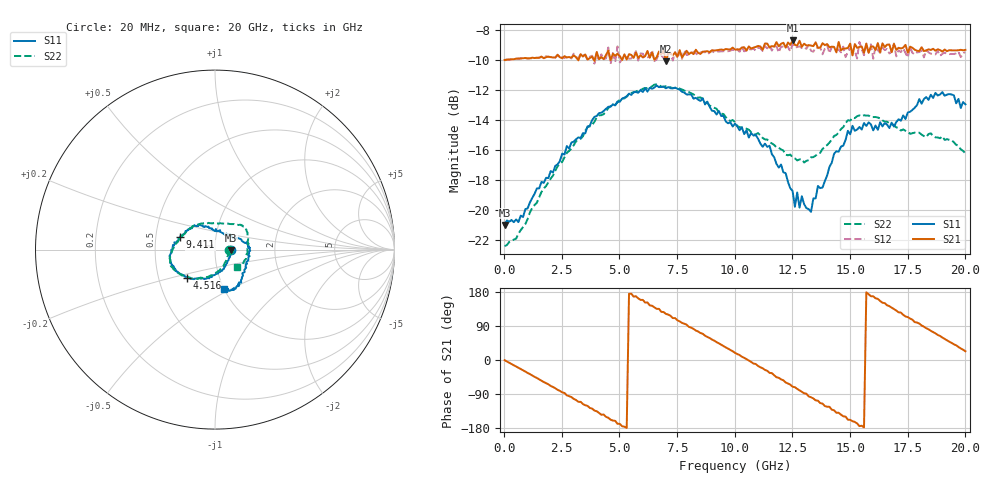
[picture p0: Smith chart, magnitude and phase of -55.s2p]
!Agilent Technologies,N5230A,US43500223,A.07.50.48
!Agilent N5230A: A.07.50.48
!Date: Saturday, October 10, 2015 17:03:50
!Correction: S11(Full 2 Port(1,2))
!S21(Full 2 Port(1,2))
!S12(Full 2 Port(1,2))
!S22(Full 2 Port(1,2))
!S2P File: Measurements: S11, S21, S12, S22:
# Hz S  RI  R 50
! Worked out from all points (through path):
!   201 points, 20 MHz to 20 GHz, reference 50 ohm
!   highest |S21| = -8.68 dB at 12.51 GHz (marker M1); lowest = -10.1 dB at 7.013 GHz (marker M2)
!   group delay of S21, straight-line fit = 96.8 ps
!   lowest |S11| = -21.0 dB at 20 MHz (marker M3), VSWR 1.20, Z = 59.8 - j0.339 ohm
!   |S11| at or under -10 dB: start of sweep to end of sweep
!   |S22| runs from -22.4 to -11.6 dB; largest |S21 - S12| = 0.034
!   S11 on the Smith chart (normalised r, x): 20 MHz: 1.20, -0.01; 4.516 GHz: 0.70, -0.23; 9.411 GHz: 0.67, +0.10; 20 GHz: 1.00, -0.46
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2e7  0.0892 -0.00281  0.3171 -0.00319  0.316 -0.00303  0.0758 -0.00311
1.8182e9  0.0285 -0.1251  0.1564 -0.2835  0.1554 -0.2872  0.0192 -0.1189
3.4166e9  -0.0786 -0.1627  -0.1436 -0.2921  -0.155 -0.2898  -0.0822 -0.1563
4.5155e9  -0.1551 -0.1579  -0.302 -0.1575  -0.3102 -0.1603  -0.1563 -0.1535
4.6154e9  -0.1619 -0.1509  -0.2926 -0.1219  -0.2871 -0.109  -0.1603 -0.1543
5.7143e9  -0.2166 -0.1205  -0.3285 0.0687  -0.3322 0.0691  -0.216 -0.1235
6.7133e9  -0.2477 -0.0698  -0.2394 0.2389  -0.2319 0.2411  -0.2459 -0.0903
7.013e9  -0.2485 -0.0579  -0.1649 0.2674  -0.1692 0.2797  -0.249 -0.0722
8.3117e9  -0.2365 0.0153  0.0729 0.3351  0.0835 0.3234  -0.2406 -0.011
9.4106e9  -0.1947 0.068  0.2621 0.2221  0.2635 0.2131  -0.2038 0.0506
1.001e10  -0.1641 0.1041  0.3249 0.111  0.3233 0.1025  -0.1787 0.0816
1.14086e10  -0.0912 0.1348  0.3157 -0.1717  0.2967 -0.1791  -0.1009 0.1393
1.25075e10  -0.0186 0.1145  0.1229 -0.3472  0.1184 -0.3383  -0.0297 0.1471
1.26074e10  0.00134 0.1026  0.1113 -0.3382  0.089 -0.3373  -0.0252 0.1468
1.34066e10  0.0636 0.0891  -0.0702 -0.3456  -0.0718 -0.33  0.0369 0.1457
1.45055e10  0.1486 0.0496  -0.2758 -0.2376  -0.2603 -0.2242  0.118 0.1382
1.53047e10  0.185 0.0164  -0.3397 -0.0759  -0.3134 -0.0682  0.1608 0.1287
1.54046e10  0.1885 0.0198  -0.3488 -0.034  -0.3613 -0.0447  0.1642 0.1263
1.67033e10  0.1743 -0.0704  -0.2814 0.2197  -0.2563 0.2131  0.1837 0.0671
1.74026e10  0.1521 -0.1322  -0.1503 0.3227  -0.1334 0.3065  0.1831 0.0192
1.83017e10  0.1366 -0.1953  0.0357 0.3392  0.0367 0.3397  0.1712 -0.038
2e10  0.0515 -0.2196  0.3152 0.1343  0.3139 0.1218  0.1216 -0.0955
